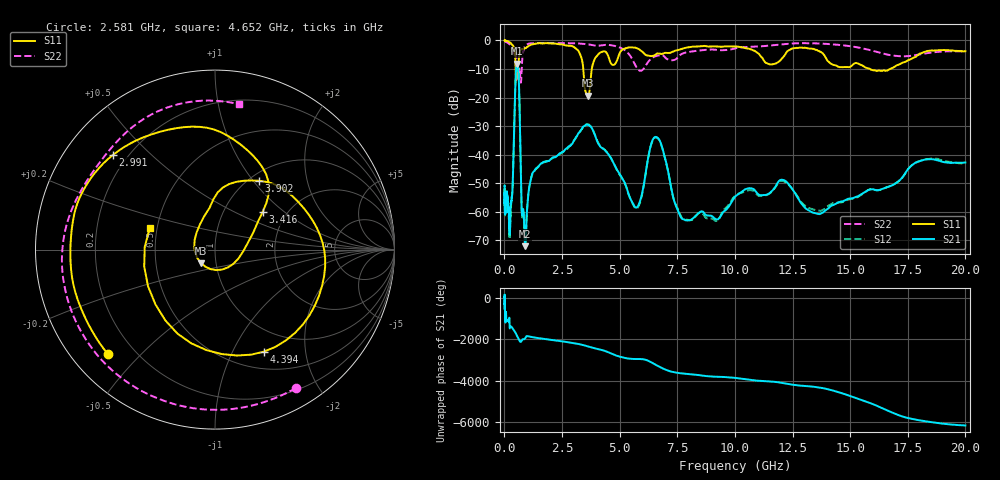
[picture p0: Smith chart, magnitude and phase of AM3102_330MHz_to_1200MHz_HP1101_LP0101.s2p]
! Date/Time: Tue, Sep 11, 2018 5:22 PM
! Network Analyzer: Agilent Technologies E8362B Rev: A.07.50.63
! Sweep from 0.010 to 20.000 GHz, 1601 Points, Sweep Type: LOG
! Power Supply: 4.949 V, 0.001 A
# Hz S DB R 50
!freq MagS11 AngS11 MagS21 AngS21 MagS12 AngS12 MagS22 AngS22
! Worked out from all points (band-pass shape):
!   1601 points, 10 MHz to 20 GHz, reference 50 ohm
!   highest |S21| = -8.17 dB at 561.8 MHz (marker M1); lowest = -72.0 dB at 907.7 MHz (marker M2)
!   |S21| within 3 dB of the highest: 499.8 MHz to 610.8 MHz (111 MHz wide, 20 % of centre)
!   lowest |S11| = -19.3 dB at 3.617 GHz (marker M3), VSWR 1.24, Z = 42.3 - j6.46 ohm
!   |S11| at or under -10 dB: 486.9 MHz to 557.4 MHz (70.5 MHz wide, 13.5 % of centre); 3.422 GHz to 3.791 GHz (368.9 MHz wide, 10.2 % of centre); 15.86 GHz to 16.74 GHz (880.6 MHz wide, 5.4 % of centre)
!   |S22| runs from -14.8 to -0.2 dB; largest |S21 - S12| = 0.0048
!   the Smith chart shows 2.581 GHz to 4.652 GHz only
!   S11 on the Smith chart (normalised r, x): 2.581 GHz: 0.11, -0.40; 2.991 GHz: 0.15, +0.39; 3.416 GHz: 1.52, +0.72; 3.902 GHz: 1.10, +1.07; 4.394 GHz: 0.71, -1.33; 4.652 GHz: 0.46, +0.13
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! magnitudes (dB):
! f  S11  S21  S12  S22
! 10 MHz  0.0  -50.8  -57.9  -0.2
! 35.55 MHz  -0.1  -59.1  -57.9  -0.3
! 126.4 MHz  -0.2  -54.5  -55.6  -0.8
! 237.7 MHz  -0.7  -67.6  -69.1  -1.4
! 357.7 MHz  -1.7  -51.0  -51.6  -4.0
! 447.2 MHz  -3.6  -23.4  -23.4  -4.1
! 561.8 MHz  -9.9  -8.2  -8.2  -9.5
! 638.6 MHz  -5.5  -17.0  -17.0  -10.1
! 754.2 MHz  -3.0  -59.7  -60.6  -9.6
! 907.7 MHz  -2.8  -72.0  -70.6  -1.9
! 1.59 GHz  -1.0  -43.1  -43.1  -0.9
! 2.581 GHz  -1.6  -38.8  -38.8  -1.0
! 2.991 GHz  -2.2  -35.4  -35.3  -1.0
! 3.416 GHz  -9.4  -30.2  -30.5  -1.2
! 3.617 GHz  -19.3  -29.5  -29.3  -1.4
! 3.902 GHz  -6.8  -32.5  -32.5  -1.8
! 4.394 GHz  -4.0  -38.7  -38.6  -1.6
! 4.652 GHz  -8.3  -41.6  -41.7  -1.7
! 5.652 GHz  -2.5  -58.2  -58.5  -8.2
! 6.58 GHz  -4.8  -33.8  -34.0  -5.5
! 7.92 GHz  -2.5  -63.0  -62.7  -4.2
! 20 GHz  -3.8  -42.7  -43.2  -3.8
